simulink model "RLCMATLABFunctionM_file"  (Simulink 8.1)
settings: Solver=ode23t  StartTime=0.0  StopTime=100  RelTol=1e-3
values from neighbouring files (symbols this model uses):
  Kd1 = K2    (= 0.04)    [MotorDCParam.m]
  Kd2 = 1/1000    (= 0.001)    [MotorDCParam.m]
  U = 5    [MotorDCParam.m]
undefined symbols (not defined in the file or in its folder): C, K, L, R

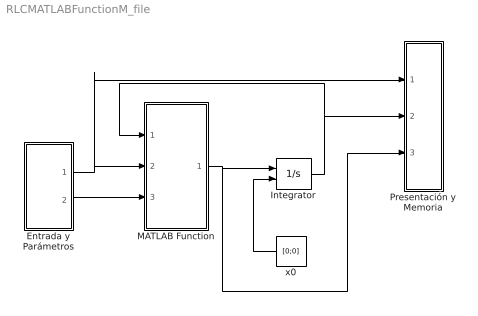
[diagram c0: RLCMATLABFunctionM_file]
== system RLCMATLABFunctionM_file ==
  Entrada y Parámetros : Subsystem
  Integrator : Integrator  InitialConditionSource=external  InitialCondition=[0;0]
  MATLAB Function : MATLAB Function  TreatAsAtomicUnit=on
  Presentación y Memoria : Subsystem
  x0 : Constant  Value=[0;0]
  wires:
  MATLAB Function/1(dx) -> Presentación y Memoria/3(dx), Integrator/1
  Integrator/1 -> MATLAB Function/1(x), Presentación y Memoria/2(x)
  x0/1 -> Integrator/2
  Entrada y Parámetros/1(u) -> Presentación y Memoria/1(u), MATLAB Function/2(u)
  Entrada y Parámetros/2(params) -> MATLAB Function/3(params)

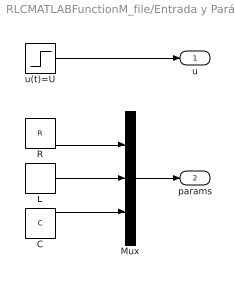
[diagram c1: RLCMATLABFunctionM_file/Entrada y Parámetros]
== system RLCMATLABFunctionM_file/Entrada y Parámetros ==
  C : Constant  Value=C
  L : Constant  Value=L
  Mux : Mux  Inputs=3
  R : Constant  Value=R
  u(t)=U : Step  Time=0  After=U  SampleTime=0
  u : Outport
  params : Outport  Port=2
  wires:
  u(t)=U/1 -> u/1
  R/1 -> Mux/1
  L/1 -> Mux/2
  C/1 -> Mux/3
  Mux/1 -> params/1

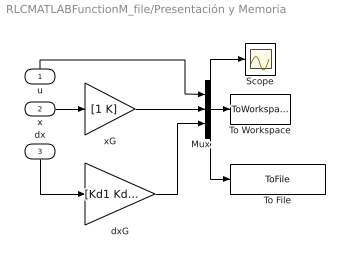
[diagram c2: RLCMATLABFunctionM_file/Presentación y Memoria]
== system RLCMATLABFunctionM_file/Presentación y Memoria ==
  u : Inport
  x : Inport  Port=2
  dx : Inport  Port=3
  Mux : Mux  Inputs=3
  Scope : Scope
  To File : ToFile  Filename=RLCFunction.mat  SaveFormat=Timeseries
  To Workspace : ToWorkspace  VariableName=RLC  SampleTime=-1
  dxG : Gain  Gain=[Kd1 Kd2]
  xG : Gain  Gain=[1 K]
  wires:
  x/1 -> xG/1
  u/1 -> Mux/1
  xG/1 -> Mux/2
  Mux/1 -> To File/1, Scope/1, To Workspace/1
  dxG/1 -> Mux/3
  dx/1 -> dxG/1

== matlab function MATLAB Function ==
function dx  = RLCState(x,u,params)
%#codegen
% x1=v_C; x2=i_L
R=params(1);
L=params(2);
C=params(3);
A=[0 1/C;-1/L -R/L];
B=[0; 1/L];
dx = A*x +B*u;
end
